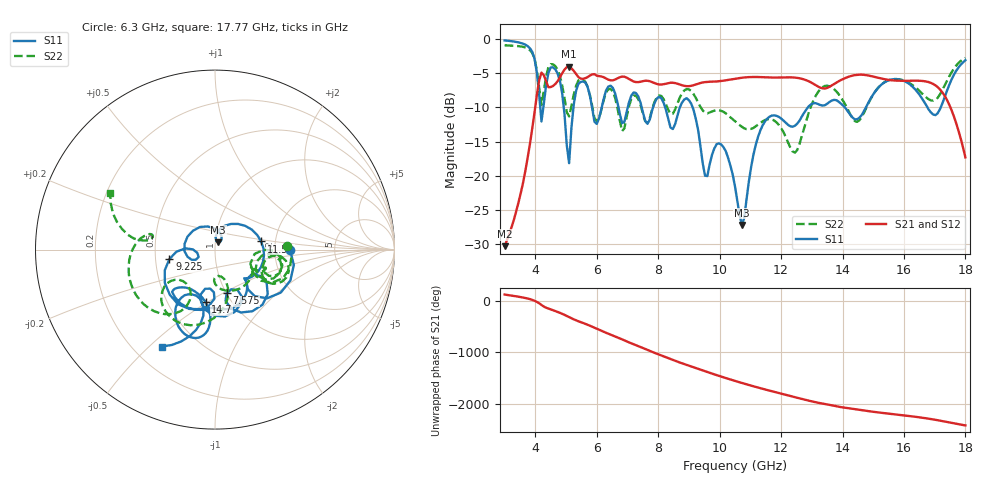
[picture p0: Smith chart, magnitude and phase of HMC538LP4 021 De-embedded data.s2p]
! Chelmsford, MA 01824
! http://www.hittite.com
! Tel: 978-250-3343
! Fax: 978-250-3373
! Device  :  HMC538LP4
! Description:  600 Analog Phase Shifter
! Frequency  :  6.0 GHz - 15.0 GHz
! Package  :  LP4  - 4x4 mm Quad Flatpack No-Lead (QFN) Plastic Package: 24 pin
! Ports  :  2 RF, 1 DC
!  Pin  3  = Rfin  = Port 1
!  Pin  16  = Rfout = Port 2
!  pin  21  = vCTL
! Voltages:  VCTL  = 0 to 5.0 Volts
! Currents :  Vb(V)  Vd(V)  Ib(mA)  Id(mA)
!  0.00  2.10  0.000000	0.475931
! Data:  The device was measured on evaluation board 111296-1.
!  Data was collected using a calibrated network analyzer.
!  The evaluation circuit board was modeled and simulated.This was use
!  to removed the evaluation board circuit from the measured data.
!  The reference plane is the center of the package pin.
! Misc:  Lot #
!Date Measured:  03 - 11 -2009
! Date:  03 - 17 -2009
! Note:
!  Hittite Microwave supplies this data as a sample of measured data at the
!  package pin for this package product.  Your particular data for this product
!  may vary.
!  Data was taken at 25 degrees C.
!  Hittite Microwave reserves the right to change this data at anytime.
# MHz S MA R 50
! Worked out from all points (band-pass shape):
!   201 points, 3 GHz to 18 GHz, reference 50 ohm
!   highest |S21| = -4.07 dB at 5.1 GHz (marker M1); lowest = -30.2 dB at 3 GHz (marker M2)
!   |S21| within 3 dB of the highest: 4.468 GHz to 13.24 GHz (8.773 GHz wide, 99.1 % of centre); 13.55 GHz to 17.1 GHz (3.544 GHz wide, 23.1 % of centre)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
!   lowest |S11| = -27.2 dB at 10.72 GHz (marker M3), VSWR 1.09, Z = 51.7 + j4.14 ohm
!   |S11| at or under -10 dB: 8.225 GHz to 8.706 GHz (481 MHz wide, 5.68 % of centre); 9.119 GHz to 12.88 GHz (3.758 GHz wide, 34.2 % of centre); 14.07 GHz to 14.76 GHz (693.6 MHz wide, 4.81 % of centre)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
!   |S22| runs from -16.6 to -1.0 dB; largest |S21 - S12| = 0.007
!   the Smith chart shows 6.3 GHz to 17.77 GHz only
!   S11 on the Smith chart (normalised r, x): 6.3 GHz: 2.43, +0.00; 7.575 GHz: 1.00, -0.52; 9.225 GHz: 0.59, -0.07; 11.55 GHz: 1.68, +0.16; 14.7 GHz: 0.76, -0.49; 17.77 GHz: 0.31, -0.55
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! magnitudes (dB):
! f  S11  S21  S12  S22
! 3 GHz  -0.3  -30.2  -30.3  -1.0
! 3.9 GHz  -1.9  -13.1  -13.0  -2.1
! 4.2 GHz  -12.1  -5.0  -5.0  -9.7
! 4.65 GHz  -4.5  -6.6  -6.6  -4.0
! 5.1 GHz  -18.2  -4.1  -4.1  -11.3
! 5.55 GHz  -6.2  -5.9  -5.9  -6.0
! 6.3 GHz  -7.6  -5.8  -5.8  -7.9
! 7.575 GHz  -12.0  -6.1  -6.2  -12.0
! 8.025 GHz  -8.5  -6.7  -6.7  -8.3
! 9.225 GHz  -11.7  -6.7  -6.7  -8.6
! 9.525 GHz  -20.0  -6.3  -6.4  -10.8
! 9.975 GHz  -15.3  -6.2  -6.2  -10.4
! 10.5 GHz  -21.6  -5.8  -5.9  -12.1
! 10.72 GHz  -27.2  -5.7  -5.7  -12.9
! 11.55 GHz  -11.7  -5.7  -5.7  -11.8
! 12.45 GHz  -12.7  -5.7  -5.7  -16.6
! 13.05 GHz  -9.4  -6.6  -6.6  -9.1
! 14.7 GHz  -10.5  -5.3  -5.3  -10.8
! 15.53 GHz  -6.0  -6.0  -6.1  -6.0
! 17.02 GHz  -11.2  -6.8  -6.8  -8.9
! 17.77 GHz  -4.2  -13.4  -13.5  -3.6
! 18 GHz  -3.2  -17.3  -17.3  -2.8
